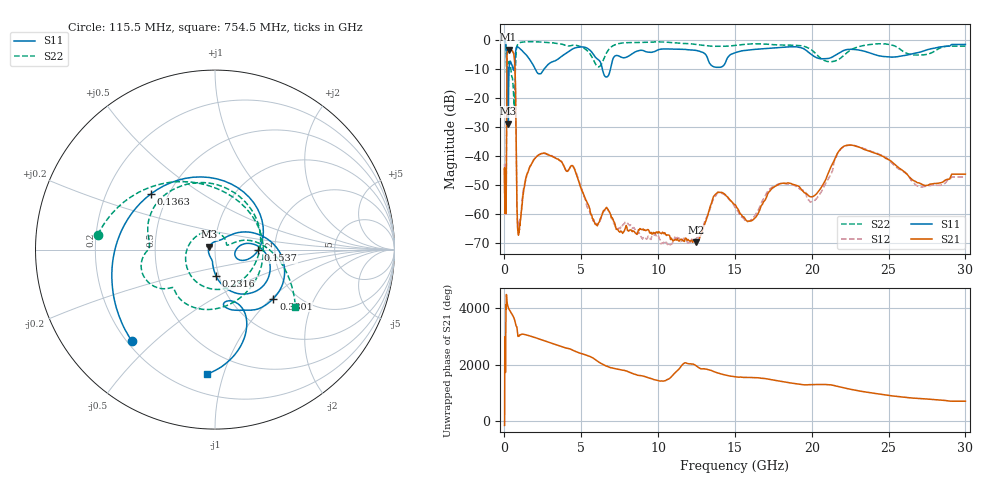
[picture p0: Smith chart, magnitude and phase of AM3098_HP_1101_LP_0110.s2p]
! Date/Time: Thu, Feb 28, 2019 8:45 AM
! Network Analyzer: Agilent Technologies E8364B Rev: A.07.50.67
! Sweep from 0.010 to 30.000 GHz, 1601 Points, Sweep Type: LOG
! Power Supply: 5.022 V, 0.002 A
# Hz S DB R 50
!freq MagS11 AngS11 MagS21 AngS21 MagS12 AngS12 MagS22 AngS22
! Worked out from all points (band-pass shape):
!   1601 points, 10 MHz to 30 GHz, reference 50 ohm
!   highest |S21| = -3.44 dB at 265.1 MHz (marker M1); lowest = -69.8 dB at 12.5 GHz (marker M2)
!   |S21| within 3 dB of the highest: 158.6 MHz to 645.1 MHz (486.5 MHz wide, 121 % of centre)
!   lowest |S11| = -28.9 dB at 250.9 MHz (marker M3), VSWR 1.07, Z = 46.9 + j1.49 ohm
!   |S11| at or under -10 dB: 207.5 MHz to 303.5 MHz (96 MHz wide, 37.6 % of centre); 1.992 GHz to 2.601 GHz (608.8 MHz wide, 26.5 % of centre); 6.368 GHz to 6.907 GHz (539 MHz wide, 8.12 % of centre)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
!   |S22| runs from -23.1 to -0.5 dB; largest |S21 - S12| = 0.012
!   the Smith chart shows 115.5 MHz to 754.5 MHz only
!   S11 on the Smith chart (normalised r, x): 115.5 MHz: 0.22, -0.42; 136.3 MHz: 0.40, +0.32; 153.7 MHz: 1.63, -0.01; 231.6 MHz: 0.97, -0.29; 380.1 MHz: 1.55, -1.03; 754.5 MHz: 0.33, -0.88
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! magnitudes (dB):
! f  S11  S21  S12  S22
! 10 MHz  -0.3  -44.7  -44.8  -0.5
! 38.04 MHz  -0.3  -57.5  -55.6  -0.7
! 115.5 MHz  -3.2  -58.2  -53.1  -3.6
! 136.3 MHz  -6.5  -25.8  -25.8  -10.8
! 144.7 MHz  -8.7  -14.3  -14.2  -10.5
! 153.7 MHz  -12.4  -8.0  -7.9  -9.3
! 231.6 MHz  -16.5  -3.6  -3.6  -8.4
! 250.9 MHz  -28.9  -3.5  -3.4  -8.7
! 265.1 MHz  -19.7  -3.4  -3.4  -8.7
! 380.1 MHz  -7.4  -3.7  -3.6  -8.6
! 550.5 MHz  -9.9  -4.2  -4.2  -14.8
! 679.2 MHz  -7.2  -9.2  -9.1  -17.5
! 754.5 MHz  -3.2  -31.0  -31.0  -5.2
! 889.9 MHz  -2.6  -66.5  -65.9  -1.5
! 2.084 GHz  -11.0  -40.4  -40.4  -0.8
! 4.436 GHz  -3.2  -43.5  -43.4  -1.9
! 7.926 GHz  -6.1  -64.0  -62.9  -1.1
! 12.5 GHz  -3.7  -69.8  -68.5  -1.6
! 13.95 GHz  -9.6  -52.6  -52.8  -2.3
! 20.31 GHz  -6.2  -53.2  -54.8  -5.1
! 22.56 GHz  -3.3  -36.3  -36.4  -3.5
! 30 GHz  -1.7  -46.3  -47.3  -2.3
